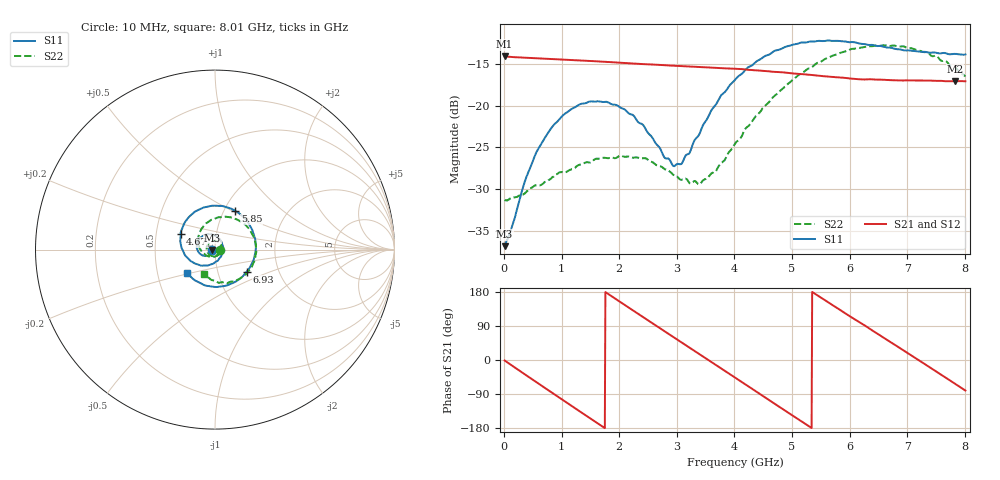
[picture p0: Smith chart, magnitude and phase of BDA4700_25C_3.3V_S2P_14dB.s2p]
!Agilent Technologies,E5071B,MY42404982,A.09.10
!Date: Mon Oct 20 18:08:54 2025
!Data & Calibration Information:
!Freq	S11:SOLT2(ON)	S21:SOLT2(ON)	S12:SOLT2(ON)	S22:SOLT2(ON)
# Hz S RI R 50
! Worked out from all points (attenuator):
!   801 points, 10 MHz to 8.01 GHz, reference 50 ohm
!   highest |S21| = -14.09 dB at 10 MHz (marker M1); lowest = -17.1 dB at 7.83 GHz (marker M2)
!   lowest |S11| = -36.8 dB at 10 MHz (marker M3), VSWR 1.03, Z = 48.6 - j0.129 ohm
!   |S11| at or under -10 dB: start of sweep to end of sweep
!   |S22| runs from -31.4 to -12.8 dB; largest |S21 - S12| = 0.0022
!   S11 on the Smith chart (normalised r, x): 10 MHz: 0.97, -0.00; 4.67 GHz: 0.67, +0.12; 5.85 GHz: 1.13, +0.52; 6.93 GHz: 1.38, -0.35; 8.01 GHz: 0.71, -0.19
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1e7  -0.0143 -0.00133  0.1974 -0.00435  0.1973 -0.00445  0.0272 -0.00102
1.5e8  -0.016 -0.011  0.1881 -0.0537  0.188 -0.0537  0.027 -0.00777
3.8e8  -0.0255 -0.0264  0.1491 -0.1241  0.149 -0.1241  0.0213 -0.0215
5.9e8  -0.042 -0.0355  0.0921 -0.169  0.0921 -0.169  0.0121 -0.031
1e9  -0.0825 -0.0242  -0.0438 -0.1843  -0.0439 -0.1844  -0.0197 -0.0349
1.35e9  -0.1021 0.0124  -0.1412 -0.1221  -0.1412 -0.1223  -0.0425 -0.0134
1.71e9  -0.0874 0.0589  -0.1832 -0.0137  -0.1833 -0.0136  -0.045 0.0188
2.07e9  -0.0437 0.0854  -0.1529 0.0961  -0.153 0.0961  -0.0231 0.0439
2.68e9  0.0359 0.0445  0.0103 0.1755  0.0101 0.1754  0.0285 0.033
2.94e9  0.0435 0.002  0.0851 0.1515  0.085 0.1512  0.0368 0.0117
3.08e9  0.0389 -0.0223  0.119 0.1254  0.1178 0.1262  0.0359 -0.00229
3.41e9  0.000821 -0.0699  0.1657 0.0407  0.1659 0.0407  0.018 -0.0291
4.01e9  -0.1244 -0.0702  0.115 -0.1205  0.1152 -0.1202  -0.0496 -0.0321
4.67e9  -0.1918 0.0867  -0.0615 -0.1475  -0.0612 -0.148  -0.0943 0.0612
5.35e9  -0.0539 0.2366  -0.1527 0.00101  -0.1527 8.52e-05  -0.00456 0.1706
5.85e9  0.1139 0.2154  -0.096 0.112  -0.0956 0.112  0.1245 0.1667
6.26e9  0.2081 0.1072  -0.00325 0.1436  -0.00122 0.1435  0.2078 0.0851
6.68e9  0.2187 -0.0431  0.0913 0.1094  0.0918 0.1093  0.2257 -0.0334
6.93e9  0.1774 -0.1221  0.1273 0.0621  0.1277 0.0615  0.2024 -0.1031
7.36e9  0.0471 -0.2032  0.1358 -0.0396  0.1359 -0.0395  0.1078 -0.1784
7.83e9  -0.1126 -0.1707  0.065 -0.1241  0.0647 -0.1243  -0.0213 -0.1685
8.01e9  -0.1576 -0.1281  0.023 -0.1384  0.0235 -0.1384  -0.0589 -0.1376
